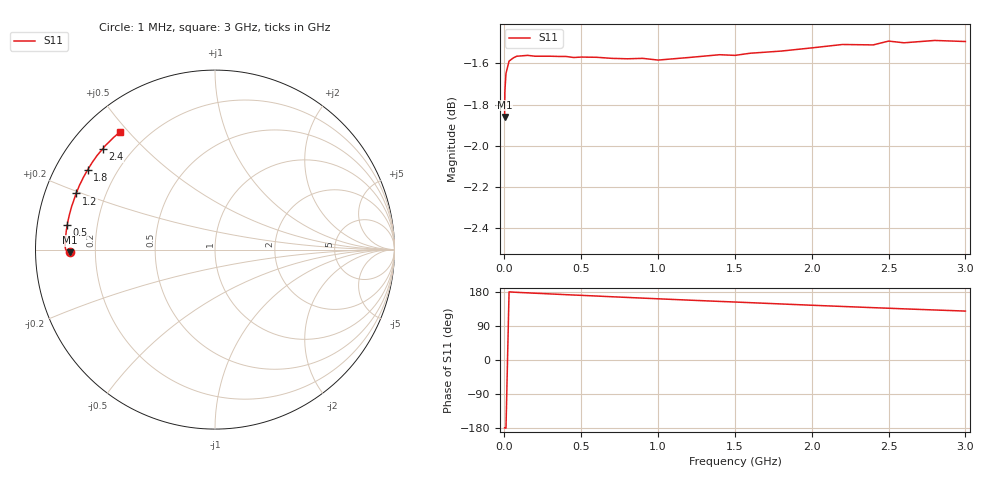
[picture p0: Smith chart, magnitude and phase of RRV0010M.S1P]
! SIEMENS Small Signal Semiconductors
! BA595
! Si PIN Diode in SOD323
! IF = 10 mA
! S-Parameters:  July  1992
# GHz  S  MA  R  50
!  f  S11
! GHz  MAG  ANG
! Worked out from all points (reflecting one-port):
!   33 points, 1 MHz to 3 GHz, reference 50 ohm
!   lowest |S11| = -1.9 dB at 1 MHz (marker M1), VSWR 9.37, Z = 5.33 - j0.475 ohm
!   phase of S11 starts at -179 deg and turns -52 deg over the sweep
!   S11 on the Smith chart (normalised r, x): 1 MHz: 0.11, -0.01; 500 MHz: 0.09, +0.08; 1.2 GHz: 0.09, +0.19; 1.8 GHz: 0.10, +0.29; 2.4 GHz: 0.10, +0.38; 3 GHz: 0.11, +0.47
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0.001  0.8072 -178.9
0.003  0.8192 -179.1
0.01  0.8271 -179.6
0.03  0.8328 179.8
0.05  0.8339 179.3
0.08  0.8351 178.6
0.15  0.8355 177.2
0.2  0.8351 176.2
0.25  0.8351 175.3
0.3  0.8351 174.3
0.4  0.835 172.4
0.5  0.8347 170.6
0.6  0.8346 168.8
0.7  0.8341 166.9
0.8  0.8339 165.1
0.9  0.8341 163.3
1.2  0.8345 158.0
1.4  0.8358 154.6
1.5  0.8355 153.0
1.6  0.8365 151.3
1.8  0.8375 147.9
2  0.839 144.5
2.2  0.8406 141.3
2.4  0.8404 138.1
2.5  0.8422 136.6
2.6  0.8414 135.0
2.8  0.8425 132.0
3  0.842 129.1
